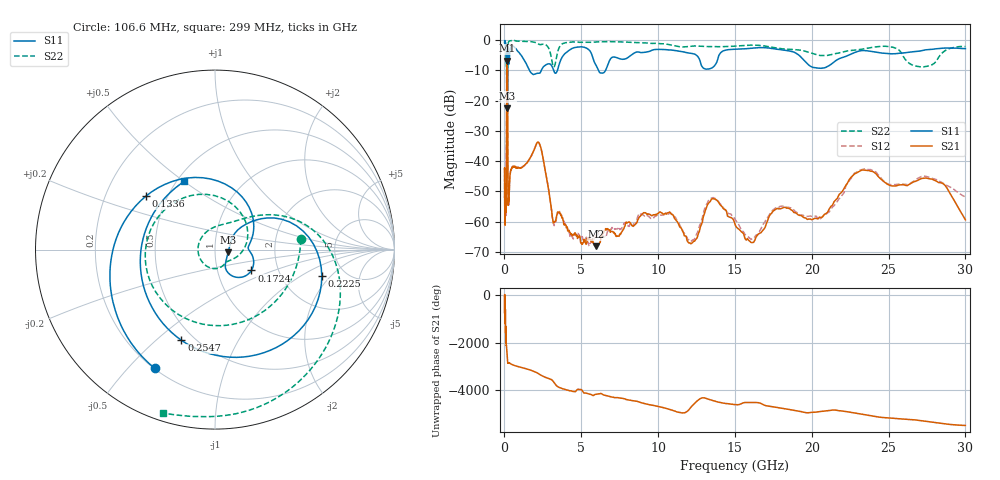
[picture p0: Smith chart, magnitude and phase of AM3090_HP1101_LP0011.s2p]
! Date/Time: Thu, Feb 28, 2019 2:07 PM
! Network Analyzer: Agilent Technologies E8364B Rev: A.07.50.67
! Sweep from 0.010 to 30.000 GHz, 1601 Points, Sweep Type: LOG
! Power Supply: 5.022 V, 0.002 A
# Hz S DB R 50
!freq MagS11 AngS11 MagS21 AngS21 MagS12 AngS12 MagS22 AngS22
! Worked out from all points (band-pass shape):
!   1601 points, 10 MHz to 30 GHz, reference 50 ohm
!   highest |S21| = -6.84 dB at 169 MHz (marker M1); lowest = -68.1 dB at 5.959 GHz (marker M2)
!   |S21| within 3 dB of the highest: 149.2 MHz to 193.9 MHz (44.71 MHz wide, 26.1 % of centre)
!   lowest |S11| = -22.5 dB at 195.4 MHz (marker M3), VSWR 1.16, Z = 57.9 - j1.78 ohm
!   |S11| at or under -10 dB: 1.624 GHz to 2.399 GHz (775.6 MHz wide, 38.6 % of centre); 3.204 GHz to 3.451 GHz (247.1 MHz wide, 7.43 % of centre); 6.112 GHz to 6.584 GHz (472.3 MHz wide, 7.44 % of centre)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
!   |S22| runs from -20.5 to -0.2 dB; largest |S21 - S12| = 0.013
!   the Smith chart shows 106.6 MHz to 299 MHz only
!   S11 on the Smith chart (normalised r, x): 106.6 MHz: 0.20, -0.60; 133.6 MHz: 0.38, +0.30; 172.4 MHz: 1.46, -0.36; 222.5 MHz: 3.37, -1.58; 254.7 MHz: 0.43, -0.61; 299 MHz: 0.55, +0.50
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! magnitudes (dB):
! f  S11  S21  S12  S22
! 10 MHz  -0.2  -42.7  -52.0  -0.6
! 38.04 MHz  -0.4  -59.4  -56.2  -1.3
! 49.84 MHz  -0.6  -47.6  -48.6  -1.3
! 106.6 MHz  -2.6  -55.9  -55.7  -6.4
! 133.6 MHz  -6.3  -27.7  -27.6  -8.6
! 144.7 MHz  -10.4  -12.9  -12.9  -13.3
! 169 MHz  -12.8  -6.8  -6.8  -19.5
! 172.4 MHz  -12.6  -6.9  -6.9  -19.8
! 195.4 MHz  -22.5  -10.5  -10.4  -14.9
! 222.5 MHz  -4.3  -47.2  -46.8  -2.4
! 254.7 MHz  -5.4  -53.7  -54.0  -0.8
! 299 MHz  -7.6  -52.1  -51.2  -0.4
! 550.5 MHz  -2.1  -41.8  -42.0  -0.2
! 2.084 GHz  -11.1  -34.3  -34.3  -1.0
! 3.204 GHz  -10.0  -60.4  -60.7  -8.9
! 5.959 GHz  -8.3  -68.1  -64.2  -0.7
! 7.926 GHz  -6.1  -60.2  -60.9  -0.7
! 12.19 GHz  -4.4  -67.1  -66.3  -2.0
! 13.74 GHz  -8.0  -52.7  -52.4  -2.2
! 16.21 GHz  -2.7  -66.9  -65.6  -1.7
! 23.48 GHz  -3.5  -43.0  -42.6  -2.9
! 30 GHz  -2.9  -59.4  -51.9  -2.2
